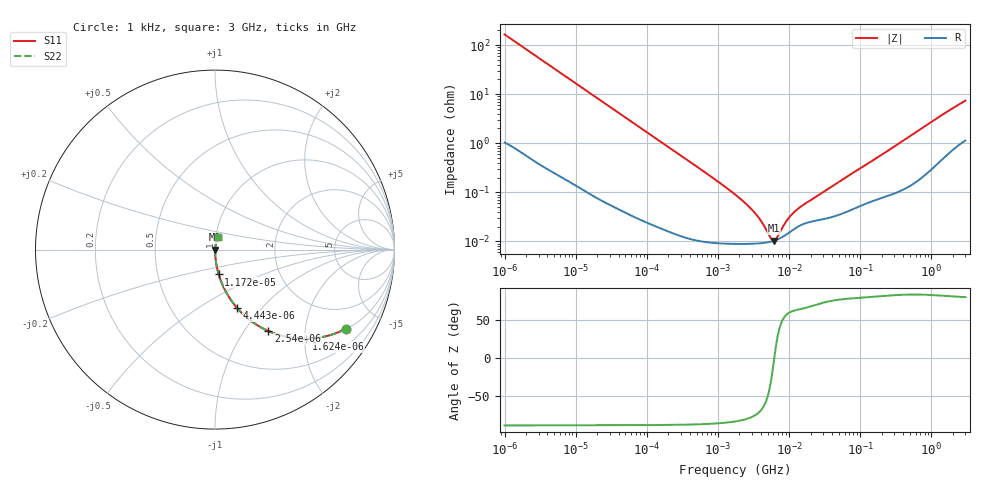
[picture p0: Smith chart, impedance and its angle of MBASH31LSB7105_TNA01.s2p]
! MBASH31LSB7105_TNA01  S-PARAMETER MODEL  ( Standard Model )
! Model Generated by TAIYO YUDEN Corporation (http://www.ty-top.com)
! Version 1.0
! TAIYO YUDEN Control No. 220601
! Copyright(c) 2013 TAIYO YUDEN CO.,LTD. All Rights Reserved.
! Product Description (link to TY-COMPAS)
! https://ds.yuden.co.jp/TYCOMPAS/or/detail?pn=MBASH31LSB7105KTNA01&u=M
! Products Name : Multilayer Ceramic Capacitors
! Characteristics :
!  Capacitance : 1 [uF] , Rated Voltage : 100 [V] , TCC : X7R
!  Case Size : 3.2 x 1.6 / 0.126 x 0.063 [mm/inch] , Thickness : 1.6 / 0.063 [mm/inch]
!  (Conditions: Temperature = 25 [degC] , DC Bias Voltage = 0 [V])
! External Node Assignments :
!  1  o---| |---o  2
! GND o---------o GND
! Frequency Range : 1kHz  -  3GHz  [ 401 STEP ]
# MHZ S RI R 50
! Freq[MHz].  S11 Real  S11 Imag  S21 Real  S21 Imag  S12 Real  S12 Imag  S22 Real  S22 Imag
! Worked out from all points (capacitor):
!   401 points, 1 kHz to 3 GHz, reference 50 ohm
!   read as one part in series: C = 969 nF near 1.077 kHz
!   lowest |Z| = 10.4 mohm at 6.153 MHz (marker M1)
!   series resonance near 6.164 MHz, so ESL is about 690 pH
!   S11 on the Smith chart (normalised r, x): 1 kHz: 1.02, -3.28; 1.624 kHz: 1.01, -2.02; 2.54 kHz: 1.01, -1.30; 4.443 kHz: 1.01, -0.74; 11.71 kHz: 1.00, -0.28; 3 GHz: 1.02, +0.15
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0.001  0.7276 -0.4421  0.2724 0.4421  0.2724 0.4421  0.7276 -0.4421
0.001624  0.506 -0.4966  0.494 0.4966  0.494 0.4966  0.506 -0.4966
0.00254  0.2972 -0.4536  0.7028 0.4536  0.7028 0.4536  0.2972 -0.4536
0.004443  0.1231 -0.3249  0.8769 0.3249  0.8769 0.3249  0.1231 -0.3249
0.006696  0.0591 -0.2319  0.9409 0.2319  0.9409 0.2319  0.0591 -0.2319
0.011715  0.0208 -0.1385  0.9792 0.1385  0.9792 0.1385  0.0208 -0.1385
0.01216  0.0194 -0.1336  0.9806 0.1336  0.9806 0.1336  0.0194 -0.1336
0.033275  0.00302 -0.0499  0.997 0.0499  0.997 0.0499  0.00302 -0.0499
0.147855  0.00032 -0.0114  0.9997 0.0114  0.9997 0.0114  0.00032 -0.0114
1.732051  9.02e-05 -0.000905  0.9999 0.000905  0.9999 0.000905  9.02e-05 -0.000905
3.264662  9.05e-05 -0.000377  0.9999 0.000377  0.9999 0.000377  9.05e-05 -0.000377
4.083148  9.25e-05 -0.000236  0.9999 0.000236  0.9999 0.000236  9.25e-05 -0.000236
5.502215  9.91e-05 -6.35e-05  0.9999 6.35e-05  0.9999 6.35e-05  9.91e-05 -6.35e-05
6.153411  0.000104 -9.57e-07  0.9999 9.57e-07  0.9999 9.57e-07  0.000104 -9.57e-07
6.629817  0.000108 4.06e-05  0.9999 -4.06e-05  0.9999 -4.06e-05  0.000108 4.06e-05
8.606987  0.000131 0.000186  0.9999 -0.000186  0.9999 -0.000186  0.000131 0.000186
10.76485  0.000164 0.000308  0.9998 -0.000308  0.9998 -0.000308  0.000164 0.000308
13.97519  0.000209 0.000444  0.9998 -0.000444  0.9998 -0.000444  0.000209 0.000444
21.06097  0.000257 0.00068  0.9997 -0.00068  0.9997 -0.00068  0.000257 0.00068
256.0921  0.000923 0.0073  0.9991 -0.0073  0.9991 -0.0073  0.000923 0.0073
1320.929  0.00547 0.0349  0.9945 -0.0349  0.9945 -0.0349  0.00547 0.0349
3000  0.0163 0.0708  0.9837 -0.0708  0.9837 -0.0708  0.0163 0.0708
